(* Logix 5000 AddOnInstructionDefinition export B256_DEC; software revision 30.00 *)

ADD_ON_INSTRUCTION B256_DEC   (* revision 1.0 20170916, vendor Kenneth A. Fischer *)
// c1 = --c1
// Revision note:
// Rev1.0: 20170916 - Initial Release
VAR_IN_OUT
   Inp_C : DINT[22]; {required}
END_VAR
VAR
   i : DINT;
END_VAR

ROUTINE Logic   (* ladder *)
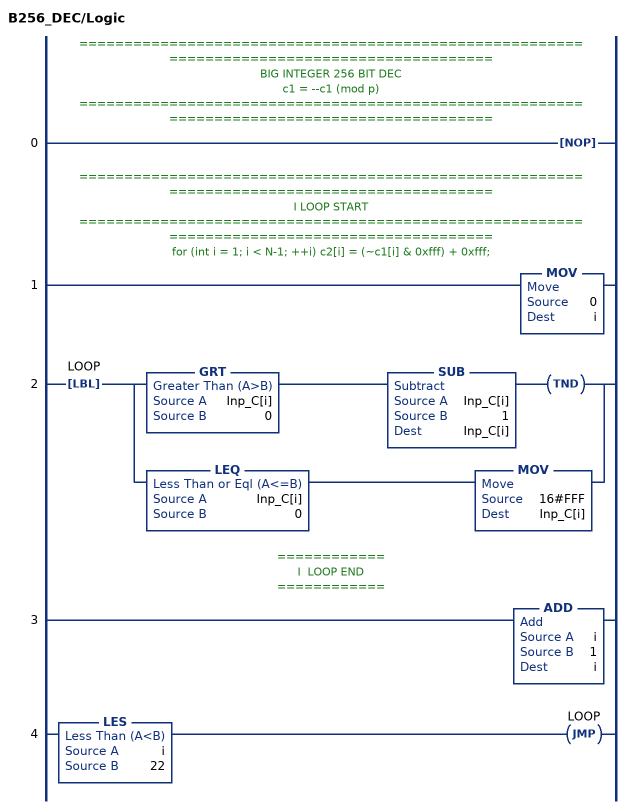
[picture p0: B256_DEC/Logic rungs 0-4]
   // ============================================================================================
   // BIG INTEGER 256 BIT DEC
   // c1 = --c1 (mod p)
   // ============================================================================================
   0: NOP();
   // ============================================================================================
   // I LOOP START
   // ============================================================================================
   // for (int i = 1; i < N-1; ++i) c2[i] = (~c1[i] & 0xfff) + 0xfff;
   1: MOV(0,i);
   2: LBL(LOOP)[GRT(Inp_C[i],0) SUB(Inp_C[i],1,Inp_C[i]) TND() ,LEQ(Inp_C[i],0) MOV(16#FFF,Inp_C[i]) ];
   // ============
   // I  LOOP END
   // ============
   3: ADD(i,1,i);
   4: LES(i,22)JMP(LOOP);
END_ROUTINE
END_ADD_ON_INSTRUCTION
